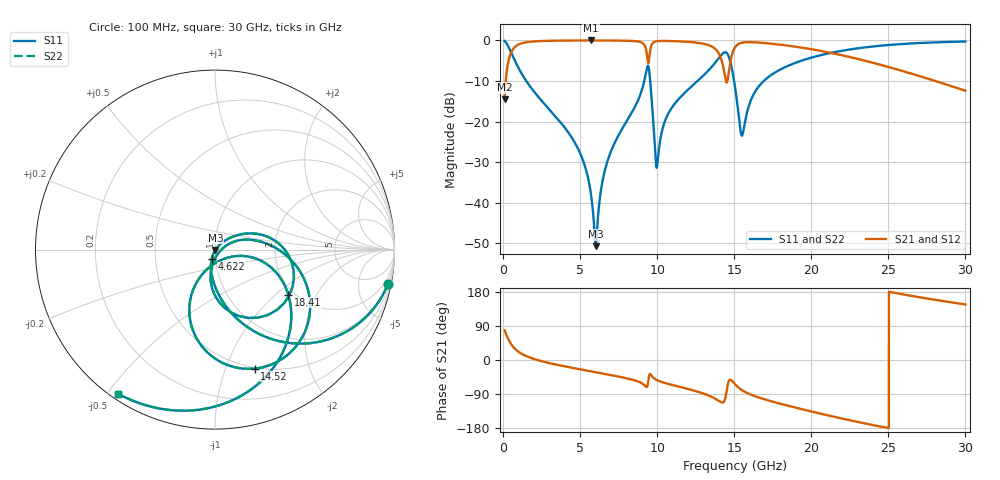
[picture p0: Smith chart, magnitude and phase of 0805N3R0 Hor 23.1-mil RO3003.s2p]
# GHz S MA R 50
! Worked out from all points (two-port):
!   3201 points, 100 MHz to 30 GHz, reference 50 ohm
!   highest |S21| = -0.03 dB at 5.706 GHz (marker M1); lowest = -14.5 dB at 100 MHz (marker M2)
!   |S21| within 3 dB of the highest: 520.2 MHz to 9.318 GHz (8.798 GHz wide, 179 % of centre); 14.89 GHz to 21.19 GHz (6.299 GHz wide, 34.9 % of centre)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
!   lowest |S11| = -50.7 dB at 6.015 GHz (marker M3), VSWR 1.01, Z = 50.3 - j0.15 ohm
!   |S11| at or under -10 dB: 1.505 GHz to 9.162 GHz (7.657 GHz wide, 144 % of centre); 9.547 GHz to 12.62 GHz (3.073 GHz wide, 27.7 % of centre); 14.99 GHz to 16.92 GHz (1.925 GHz wide, 12.1 % of centre)
!   |S22| runs from -50.7 to -0.2 dB; largest |S21 - S12| = 0
!   S11 on the Smith chart (normalised r, x): 100 MHz: 1, -10; 4.622 GHz: 0.96, -0.10; 14.52 GHz: 0.49, -1.27; 18.41 GHz: 1.87, -1.21; 30 GHz: 0.02, -0.53
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0.1  0.9822 -11.3  0.1874 78.6  0.1874 78.6  0.9822 -11.3
0.5017812  0.7206 -46.6  0.6928 43.4  0.6928 43.4  0.7206 -46.6
1.296  0.3646 -75.5  0.93 14.4  0.93 14.4  0.3646 -75.5
4.622375  0.05647 -109.3  0.9959 -21.6  0.9959 -21.6  0.05647 -109.3
5.089563  0.03717 -111.3  0.9966 -25.2  0.9966 -25.2  0.03717 -111.3
5.70625  0.01266 -107.2  0.9969 -29.9  0.9969 -29.9  0.01266 -107.2
6.014594  0.002927 -30.7  0.9969 -32.2  0.9969 -32.2  0.002927 -30.7
6.780781  0.03279 46.0  0.9958 -38.0  0.9958 -38.0  0.03279 46.0
9.340969  0.4596 -16.9  0.6581 -71.0  0.6581 -71.0  0.4596 -16.9
9.658656  0.1701 -98.3  0.8937 -42.7  0.8937 -42.7  0.1701 -98.3
10.06978  0.03829 3.1  0.9787 -54.6  0.9787 -54.6  0.03829 3.1
10.81728  0.1351 21.7  0.9808 -64.2  0.9808 -64.2  0.1351 21.7
13.15322  0.3942 -4.3  0.8949 -90.8  0.8949 -90.8  0.3942 -4.3
14.09694  0.6383 -34.2  0.6305 -110.3  0.6305 -110.3  0.6383 -34.2
14.51741  0.699 -71.5  0.3025 -79.5  0.3025 -79.5  0.699 -71.5
15.05  0.2676 -118.2  0.8196 -63.8  0.8196 -63.8  0.2676 -118.2
15.51719  0.06766 -58.4  0.9362 -79.9  0.9362 -79.9  0.06766 -58.4
16.46091  0.251 -13.0  0.9423 -97.2  0.9423 -97.2  0.251 -13.0
18.41375  0.4785 -31.5  0.8636 -119.9  0.8636 -119.9  0.4785 -31.5
20.03956  0.6152 -47.3  0.7756 -136.2  0.7756 -136.2  0.6152 -47.3
25.01978  0.8765 -90.6  0.4694 -179.9  0.4694 -179.9  0.8765 -90.6
30  0.9674 -123.9  0.2396 146.7  0.2396 146.7  0.9674 -123.9
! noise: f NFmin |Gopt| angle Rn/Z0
0.1  0.0009198  0.9342  1.263  0.003113
3.417  0.006185  0.6987  18.9  0.00391
6.743  0.0114  0.6858  35.84  0.006401
10.06  0.03395  0.8331  52.69  0.03455
13.39  0.0513  0.8556  68.33  0.05209
16.7  0.04512  0.8057  83.38  0.02717
20.03  0.03975  0.752  96.3  0.01475
23.35  0.04778  0.7672  108.9  0.0146
26.67  0.06213  0.8021  121.4  0.0162
30  0.08559  0.8452  134  0.01862
